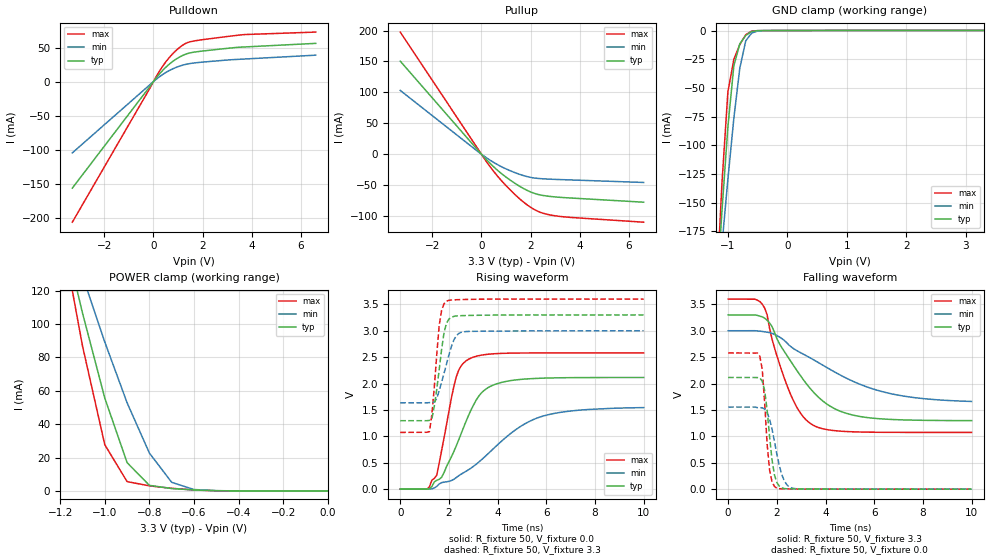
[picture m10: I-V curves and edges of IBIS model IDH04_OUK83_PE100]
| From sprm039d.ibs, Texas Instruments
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[Model]   IDH04_OUK83_PE100
| I/O with pulldown
Model_type   I/O
Vinh = 2.00
Vinl = 0.80
Enable   Active-Low
Polarity   Non-Inverting
| signals   A, GZ, Y
Vmeas = 1.5
|   typ   min   max
C_comp   2.800p   2.792p   2.860p
|   typ   min   max
[Temperature Range]   25   -40   125
|   typ   min   max
[Voltage Range]   3.30V   3.00V   3.60V
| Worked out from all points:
|   slope of the pulldown table from 0 to 0.495 V, typ, clamps not added: 23.8 ohm
|   slope of the pullup table from 0 to 0.495 V, typ, clamps not added: 24.4 ohm
|   GND clamp passes 1 mA (typ) near -0.60 V on its own axis
|   POWER clamp passes 1 mA (typ) near -0.65 V on its own axis
|   rising waveform, R_fixture 50, V_fixture 0.0: 20-80 % time 1.23ns typ, 2.52ns min, 658ps max; typ from 0 V to 2.12 V
|   falling waveform, R_fixture 50, V_fixture 3.3: 20-80 % time 1.85ns typ, 3.26ns min, 1.11ns max; typ from 3.3 V to 1.3 V
|   rising waveform, R_fixture 50, V_fixture 3.3: 20-80 % time 339ps typ, 495ps min, 267ps max; typ from 1.3 V to 3.3 V
|   falling waveform, R_fixture 50, V_fixture 0.0: 20-80 % time 300ps typ, 436ps min, 237ps max; typ from 2.12 V to 0 V
[Pulldown]
|   Voltage   I(typ)   I(min)   I(max)
-3.3V     -156.5mA   -104.8mA   -206.6mA
-200mV    -9.762mA   -6.342mA   -13.16mA
200mV     9.308mA    5.91mA     12.77mA
600mV     24.27mA    15.38mA    33.46mA
800mV     30.04mA    19mA       41.54mA
1.1V      36.8mA     23.15mA    51.22mA
1.3V      40.12mA    25.17mA    55.93mA
1.6V      42.95mA    27.12mA    59.33mA
3.5V      50.51mA    32.76mA    68.38mA
6.6V      56.15mA    38.81mA    72.73mA
[GND_clamp]
|   Voltage   I(typ)   I(min)   I(max)
-3.3V     -2.129A    -1.609A    -2.759A
-1.2V     -238.4mA   -247mA     -237.3mA
-1.1V     -157.5mA   -187.2mA   -133.3mA
-1V       -83.99mA   -129.6mA   -53.52mA
-900mV    -30.8mA    -76.5mA    -25.17mA
-800mV    -11.67mA   -32.9mA    -12.22mA
-700mV    -4.303mA   -9.006mA   -3.656mA
-600mV    -880.1uA   -2.169mA   -490.6uA
-500mV    -121uA     -404.6uA   -89.22uA
-400mV    -40.3uA    -67.11uA   -56.25uA
3.3V      100.8uA    54.12uA    177.3uA
[Pullup]
|   Voltage   I(typ)   I(min)   I(max)
-3.3V     150.6mA    103.2mA    197.6mA
-200mV    9.015mA    6.05mA     12.03mA
300mV     -12.71mA   -8.337mA   -17.25mA
900mV     -34.06mA   -21.94mA   -46.59mA
1.4V      -48.08mA   -30.44mA   -66.63mA
1.8V      -57.38mA   -35.68mA   -80.27mA
2.3V      -65.13mA   -39.22mA   -92.49mA
2.9V      -68.83mA   -40.65mA   -99.12mA
3.7V      -71.1mA    -41.8mA    -102.6mA
6.6V      -77.74mA   -45.8mA    -110.1mA
[POWER_clamp]
|   Voltage   I(typ)   I(min)   I(max)
-3.3V     1.472A     1.113A     1.907A
-1.2V     162.8mA    170.3mA    159.8mA
-1.1V     106.7mA    128.9mA    86.98mA
-1V       55.67mA    89.28mA    27.7mA
-900mV    16.96mA    52.84mA    5.593mA
-800mV    3.336mA    22.68mA    3.033mA
-700mV    1.434mA    5.139mA    1.568mA
-600mV    594uA      840.3uA    550.9uA
-500mV    140.8uA    157.5uA    81.51uA
0V        1pA        1pA        1pA
[Ramp]
|   I(typ)   I(min)   I(max)
dV/dt_r   1.269/1.229n   0.927/2.521n   1.548/0.655n
dV/dt_f   1.201/1.857n   0.803/3.256n   1.515/1.104n
[Rising Waveform]
R_fixture = 50
V_fixture = 0.0
|  pu_on
|  TIME   V(typ)   V(min)   V(max)
0s        4nV        16nV       3nV
1.1ns     259.6uV    484.4uV    1.871mV
1.5ns     168.6mV    52.49mV    266.7mV
1.7ns     224.8mV    124.5mV    733.1mV
2.3ns     818.1mV    219.1mV    2.123V
2.8ns     1.39V      366.3mV    2.459V
3.2ns     1.745V     502.2mV    2.525V
3.7ns     1.946V     711.4mV    2.559V
5.7ns     2.099V     1.36V      2.58V
10ns      2.115V     1.545V     2.58V
[Falling Waveform]
R_fixture = 50
V_fixture = 3.3
V_fixture_min = 3.0
V_fixture_max = 3.6
|  pd_on
|  TIME   V(typ)   V(min)   V(max)
0s        3.3V       3V         3.6V
1.4ns     3.263V     2.987V     3.506V
1.6ns     3.199V     2.973V     3.304V
1.8ns     3.081V     2.95V      2.846V
2.5ns     2.472V     2.728V     1.867V
3ns       2.131V     2.578V     1.423V
3.5ns     1.84V      2.452V     1.209V
4.3ns     1.542V     2.238V     1.112V
5.4ns     1.377V     1.989V     1.083V
10ns      1.298V     1.661V     1.075V
[Rising Waveform]
R_fixture = 50
V_fixture = 3.3
V_fixture_min = 3.0
V_fixture_max = 3.6
|  pd_off
|  TIME   V(typ)   V(min)   V(max)
0s        1.297V     1.636V     1.075V
1.2ns     1.303V     1.639V     1.089V
1.3ns     1.335V     1.645V     1.412V
1.4ns     1.571V     1.65V      1.933V
1.6ns     2.262V     1.864V     3.099V
1.7ns     2.649V     2.026V     3.386V
1.9ns     3.143V     2.369V     3.56V
2.2ns     3.271V     2.823V     3.585V
2.6ns     3.287V     2.979V     3.592V
10ns      3.3V       3V         3.6V
[Falling Waveform]
R_fixture = 50
V_fixture = 0.0
|  pu_off
|  TIME   V(typ)   V(min)   V(max)
0s        2.115V     1.555V     2.58V
1.3ns     2.109V     1.544V     2.519V
1.4ns     2.044V     1.541V     2.271V
1.5ns     1.871V     1.518V     1.632V
1.7ns     1.005V     1.329V     363.6mV
1.8ns     563.2mV    1.142V     144.2mV
2ns       126.4mV    664.8mV    18.55mV
2.3ns     11.94mV    165mV      6.142mV
2.7ns     5.183mV    12.42mV    3.12mV
10ns      13.99uV    80.02uV    426nV
